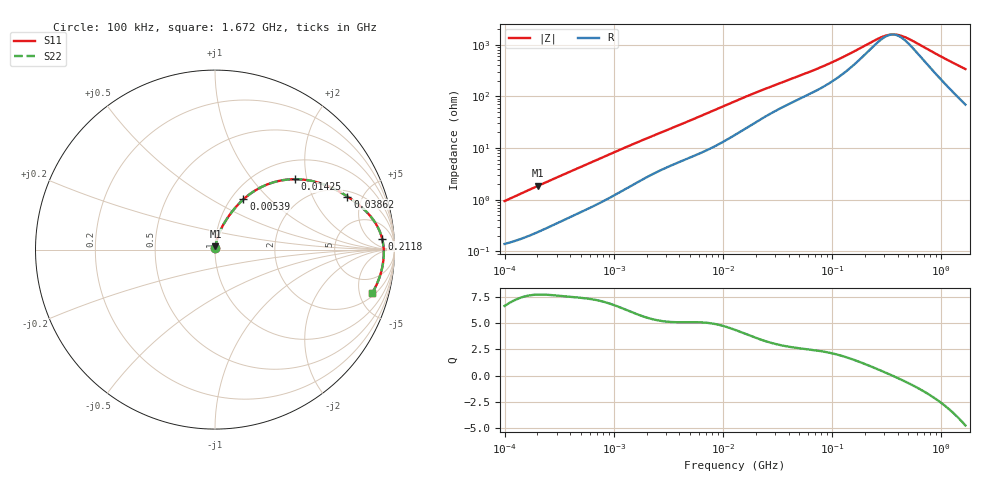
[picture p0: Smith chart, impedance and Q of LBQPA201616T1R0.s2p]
! LBQPA201616T1R0  S-PARAMETER MODEL  ( General Type )
! Model Generated by TAIYO YUDEN Corporation (http://www.ty-top.com)
! Version 1.0
! TAIYO YUDEN Control No. 191025NI43SB-FBB
! Copyright(c) 2019 TAIYO YUDEN CO.,LTD. All Rights Reserved.
! Product Description (link to TY-COMPAS)
! https://ds.yuden.co.jp/TYCOMPAS/or/detail?pn=LBQPA201616T1R0M&u=M
! Products Name : Inductors
! Characteristics :
!  Inductance : 1.0 uH , SRF(min) : 100 MHz , DC Resistance(max) : 0.13 Ohm
!  Rated Current : Saturation :1100 mA , Temp Rise : 885 mA (20 degC)
!  Case Size : 2.0 x 1.6 / 0.079 x 0.063 [mm/inch] , Thickness : 1.6 / 0.063 [mm/inch]
!  (Conditions: Temperature = 25 degC , DC Bias Current/Voltage = 0A / 0V)
! External Node Assignments :
!  1  o---GGG---o  2
! GND o---------o GND
! Frequency Range : 0.1MHz  -  1672.468556MHz  [ 402 STEP ]
# MHz S RI R 50
! Freq[MHz].  S11 Real  S11 Imag  S21 Real  S21 Imag  S12 Real  S12 Imag  S22 Real  S22 Imag
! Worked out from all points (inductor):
!   401 points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, 100 kHz to 1.672 GHz, reference 50 ohm
!   read as one part in series: L = 1.48 uH near 105 kHz
!   highest Q = 7.75 at 202.4 kHz (marker M1), where L = 1.45 uH
!   self-resonance near 356.9 MHz
!   S11 on the Smith chart (normalised r, x): 100 kHz: 1.00, +0.02; 5.39 MHz: 1.14, +0.71; 14.25 MHz: 1.41, +1.71; 38.62 MHz: 2.36, +3.78; 211.8 MHz: 15, +14; 1.672 GHz: 2.38, -6.59
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0.1  0.00148 0.0093  0.9985 -0.0093  0.9985 -0.0093  0.00148 0.0093
0.202392  0.00271 0.0183  0.9973 -0.0183  0.9973 -0.0183  0.00271 0.0183
0.509815  0.00769 0.043  0.9923 -0.043  0.9923 -0.043  0.00769 0.043
1.193868  0.0232 0.0919  0.9768 -0.0919  0.9768 -0.0919  0.0232 0.0919
2.599112  0.0658 0.1705  0.9342 -0.1705  0.9342 -0.1705  0.0658 0.1705
3.834946  0.1056 0.2246  0.8944 -0.2246  0.8944 -0.2246  0.1056 0.2246
5.389851  0.1586 0.2803  0.8414 -0.2803  0.8414 -0.2803  0.1586 0.2803
8.148346  0.2573 0.348  0.7427 -0.348  0.7427 -0.348  0.2573 0.348
12.9324  0.4116 0.3909  0.5884 -0.3909  0.5884 -0.3909  0.4116 0.3909
14.25321  0.4468 0.3923  0.5532 -0.3923  0.5532 -0.3923  0.4468 0.3923
23.74865  0.6172 0.359  0.3828 -0.359  0.3828 -0.359  0.6172 0.359
38.61951  0.7377 0.2958  0.2623 -0.2958  0.2623 -0.2958  0.7377 0.2958
65.93127  0.833 0.2214  0.167 -0.2214  0.167 -0.2214  0.833 0.2214
118.1661  0.9001 0.1375  0.0999 -0.1375  0.0999 -0.1375  0.9001 0.1375
211.7846  0.9313 0.0607  0.0687 -0.0607  0.0687 -0.0607  0.9313 0.0607
276.7176  0.9374 0.0291  0.0626 -0.0291  0.0626 -0.0291  0.9374 0.0291
336.1274  0.9397 0.00684  0.0603 -0.00684  0.0603 -0.00684  0.9397 0.00684
398.4856  0.9404 -0.0126  0.0596 0.0126  0.0596 0.0126  0.9404 -0.0126
472.4126  0.9401 -0.0326  0.0599 0.0326  0.0599 0.0326  0.9401 -0.0326
979.6553  0.9229 -0.1345  0.0771 0.1345  0.0771 0.1345  0.9229 -0.1345
1410.747  0.8966 -0.2032  0.1034 0.2032  0.1034 0.2032  0.8966 -0.2032
1672.469  0.8768 -0.2403  0.1232 0.2403  0.1232 0.2403  0.8768 -0.2403
